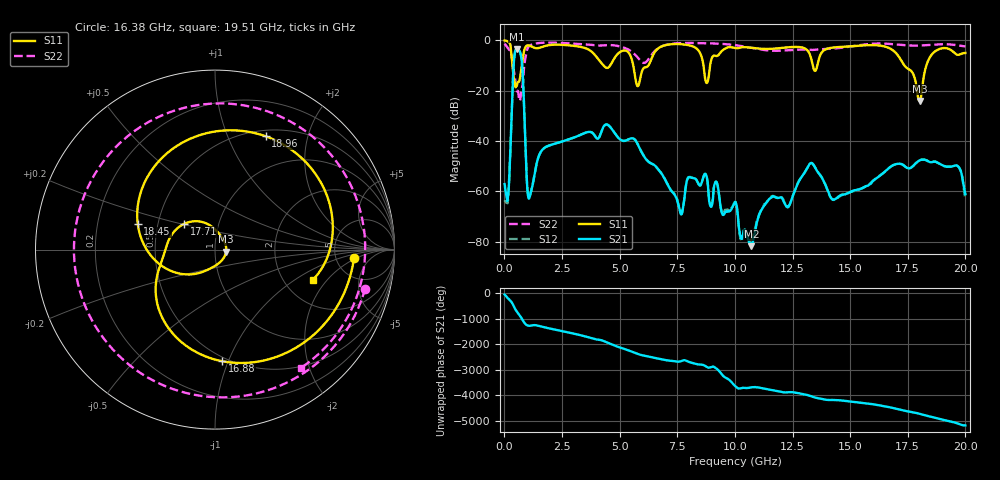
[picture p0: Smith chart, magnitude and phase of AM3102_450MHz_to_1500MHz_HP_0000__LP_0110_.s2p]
!Agilent Technologies,E8364B,MY43040894,A.07.50.67
!Agilent E8364B: A.07.50.67
!Date: Thursday, January 11, 2018 05:16:13
!Correction: S11(Full 2 Port(1,2))
!S21(Full 2 Port(1,2))
!S12(Full 2 Port(1,2))
!S22(Full 2 Port(1,2))
!S2P File: Measurements: S11, S21, S12, S22:
# Hz S  dB  R 50
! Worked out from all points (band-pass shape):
!   1601 points, 10 MHz to 20 GHz, reference 50 ohm
!   highest |S21| = -3.43 dB at 547.2 MHz (marker M1); lowest = -81.8 dB at 10.72 GHz (marker M2)
!   |S21| within 3 dB of the highest: 433.1 MHz to 727.1 MHz (294 MHz wide, 50.7 % of centre)
!   lowest |S11| = -24.1 dB at 18.01 GHz (marker M3), VSWR 1.13, Z = 56.5 - j1.28 ohm
!   |S11| at or under -10 dB: 348.2 MHz to 754.9 MHz (406.7 MHz wide, 73.7 % of centre); 5.591 GHz to 6.246 GHz (655 MHz wide, 11.1 % of centre); 17.36 GHz to 18.31 GHz (950.6 MHz wide, 5.33 % of centre)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
!   |S22| runs from -24.1 to -0.9 dB; largest |S21 - S12| = 0.0027
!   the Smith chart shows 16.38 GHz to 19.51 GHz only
!   S11 on the Smith chart (normalised r, x): 16.38 GHz: 7.45, -1.83; 16.88 GHz: 0.47, -0.95; 17.71 GHz: 0.68, +0.21; 18.45 GHz: 0.38, +0.14; 18.96 GHz: 0.57, +1.38; 19.51 GHz: 2.85, -1.43
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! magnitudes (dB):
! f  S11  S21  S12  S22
! 10 MHz  0.0  -57.1  -63.6  -1.3
! 172.4 MHz  -0.6  -60.7  -61.7  -3.4
! 547.2 MHz  -17.8  -3.4  -3.4  -20.3
! 747.1 MHz  -10.5  -7.7  -7.7  -19.7
! 1.084 GHz  -2.1  -62.7  -62.3  -2.2
! 3.346 GHz  -2.7  -37.4  -37.3  -1.5
! 5.782 GHz  -18.2  -41.2  -41.2  -6.8
! 6.682 GHz  -3.1  -51.4  -51.4  -3.1
! 8.781 GHz  -17.0  -54.4  -54.3  -1.1
! 10.01 GHz  -3.1  -64.2  -64.3  -1.9
! 10.72 GHz  -3.0  -81.8  -78.8  -3.0
! 13.34 GHz  -8.4  -48.8  -48.8  -3.8
! 14.28 GHz  -2.8  -63.3  -63.3  -3.3
! 16.38 GHz  -2.2  -53.2  -53.1  -1.3
! 16.68 GHz  -3.0  -50.8  -50.8  -1.4
! 16.88 GHz  -4.1  -49.5  -49.6  -1.6
! 17.71 GHz  -13.0  -50.1  -50.1  -2.1
! 18.01 GHz  -24.1  -47.7  -47.7  -2.1
! 18.45 GHz  -6.9  -48.4  -48.4  -1.8
! 18.96 GHz  -3.2  -49.5  -49.5  -1.6
! 19.51 GHz  -4.9  -49.8  -49.9  -1.8
! 20 GHz  -5.0  -61.1  -63.3  -2.4
